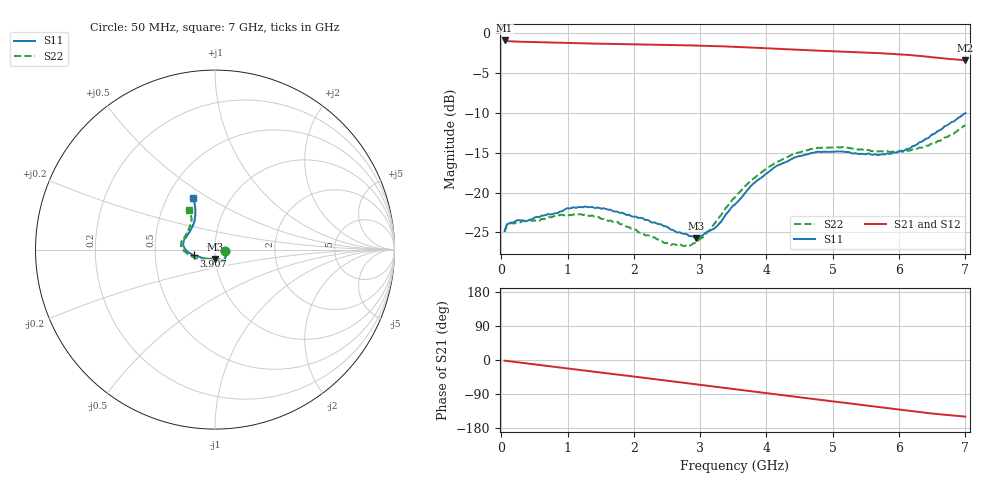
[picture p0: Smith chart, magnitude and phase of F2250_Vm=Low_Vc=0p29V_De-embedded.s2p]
! Integrated Device Technology
! Corporate Headquarters
! 6024 Silver Creek Valley Road
! San Jose, CA 95138  USA
! Phone:  1-408-284-8200
! Toll Free:  1-800-223-1366
! Webpage:  http://www.idt.com/
! Timing and RF Division
! 515 Groton Road, Suite 102
! Westford, MA 01886-6024
! Device:  F2250
! Description: Voltage Variable RF Attenuator
! Frequency:  50.0 -  6000.00 MHz
! Package:  3x3 mm Thin QFN Plastic Package: 16 pin
! Ports:  2 RF, 3 DC
!  Pin  1  = GND
!  Pin  2  = NC
!  Pin  3  = RF1  = Port 1
!  Pin  4  = NC
!  Pin  5  = GND
!  Pin  6  = GND
!  Pin  7  = GND
!  Pin  8  = GND
!  Pin  9  = NC
!  Pin 10  = RF2  = Port 2
!  Pin 11  = NC
!  Pin 12  = GND
!  Pin 13  = GND
!  Pin 14  = VCNTRL
!  Pin 15  = VDD
!  Pin 16  = VMODE
! Vcntrl:  0.290 Volts
! Vmode:  +0.000 Volts
! Vdd:  +3.30  Volts
! Current:  1.115 mA
! Data:  The device was measured on a the F2250 evaluation board which has
!  individual transmission lines to the RF pins.  Data was collected
!  using a calibrated network analyzer.  The evaluation board was
!  de-embedded using a TRL calibration technique.
!  The reference plane is the edge of the package pin.
! Misc:  SN 10
!  Action Tracker AT0258
! Date Measured:  2014-11-26
! Date:  2015-10-15  MJV
! Note:
!  Integrated Device Technology supplies this data as a sample of measured
!  data at the package pin for this product.  Your particular data for this
!  product may vary.
!  Data was taken at 25 degrees C.
!  Integrated Device Technology reserves the right to change this data at anytime.
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# GHz S dB R 50
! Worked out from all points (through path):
!   201 points, 50 MHz to 7 GHz, reference 50 ohm
!   highest |S21| = -0.95 dB at 50 MHz (marker M1); lowest = -3.4 dB at 7 GHz (marker M2)
!   group delay of S21, straight-line fit = 60 ps
!   lowest |S11| = -25.7 dB at 2.934 GHz (marker M3), VSWR 1.11, Z = 49.7 - j5.17 ohm
!   |S11| at or under -10 dB: start of sweep to end of sweep
!   |S22| runs from -26.7 to -11.6 dB; largest |S21 - S12| = 0.00034
!   S11 on the Smith chart (normalised r, x): 50 MHz: 1.12, -0.02; 3.907 GHz: 0.79, -0.05; 7 GHz: 0.67, +0.43
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0.05  -24.80 -9.4  -0.95 -1.8  -0.94 -1.8  -24.93 -9.9
0.08475  -23.98 -9.3  -1.02 -2.5  -1.02 -2.5  -24.06 -9.1
0.15425  -23.76 -11.6  -1.06 -4.0  -1.06 -4.0  -23.81 -10.9
0.57125  -23.08 -29.4  -1.16 -13.1  -1.16 -13.1  -23.53 -30.0
0.884  -22.39 -45.0  -1.23 -19.9  -1.23 -19.9  -22.80 -46.3
1.2315  -21.85 -55.1  -1.30 -27.4  -1.30 -27.4  -22.81 -59.2
1.75275  -22.39 -61.8  -1.40 -38.4  -1.39 -38.4  -23.67 -66.3
2.37825  -23.96 -62.7  -1.49 -51.8  -1.48 -51.8  -25.94 -68.3
2.552  -24.63 -66.8  -1.51 -55.6  -1.51 -55.6  -26.58 -73.9
2.83  -25.43 -81.8  -1.56 -61.7  -1.56 -61.7  -26.71 -92.8
2.93425  -25.70 -90.7  -1.58 -64.0  -1.58 -64.0  -26.34 -101.4
3.21225  -24.52 -120.1  -1.65 -70.2  -1.65 -70.2  -23.93 -127.1
3.525  -21.49 -146.9  -1.74 -77.1  -1.74 -77.1  -20.58 -146.0
3.76825  -19.14 -160.3  -1.83 -82.5  -1.83 -82.5  -18.47 -156.4
3.90725  -18.22 -164.6  -1.89 -85.5  -1.89 -85.5  -17.58 -162.5
4.1505  -16.67 -173.0  -1.99 -90.8  -1.99 -90.8  -16.20 -171.2
4.7065  -15.01 172.8  -2.20 -102.9  -2.20 -102.9  -14.55 175.8
5.15825  -14.87 162.1  -2.36 -112.6  -2.36 -112.6  -14.30 166.6
5.85325  -15.15 138.9  -2.60 -127.5  -2.61 -127.5  -14.92 151.5
6.166  -14.46 127.9  -2.77 -134.3  -2.78 -134.3  -14.74 142.6
6.444  -13.15 119.6  -2.98 -140.1  -2.98 -140.1  -14.13 133.3
7  -10.06 113.2  -3.43 -149.4  -3.43 -149.4  -11.57 123.8
